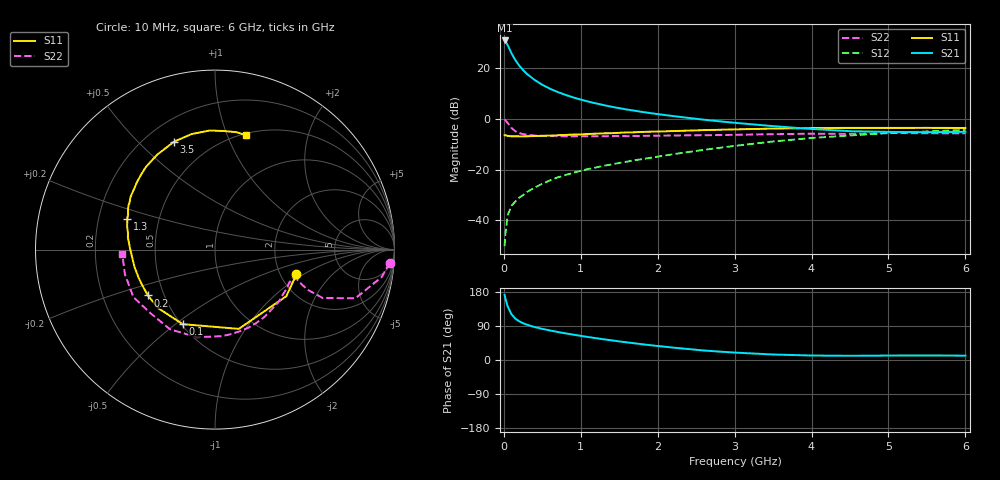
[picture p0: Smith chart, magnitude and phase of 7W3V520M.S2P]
! Infineon Technologies  Discrete & RF Semiconductors
! BFS17W
! Si NPN RF Bipolar Junction Transistor in SOT323
! VCE = 3.5 V  IC = 20 mA
! Common Emitter S-Parameters:  August  1999
# GHz  S  MA  R  50
!  f  S11  S21  S12  S22
! GHz  MAG  ANG  MAG  ANG  MAG  ANG  MAG  ANG
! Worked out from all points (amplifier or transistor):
!   36 points, 10 MHz to 6 GHz, reference 50 ohm
!   highest |S21| = 30.9 dB at 10 MHz (marker M1)
!   |S21| within 3 dB of that: start of sweep to 67.79 MHz
!   unconditionally stable (mu >= 1): 266.7 MHz to 2.291 GHz; 4.78 GHz to end of sweep
!   at 250 MHz: K = 0.98, MSG = 24.6 dB, |S12| = -30.0 dB
!   at 1.4 GHz: K = 1.19, MAG = 8.8 dB, |S12| = -18.0 dB
!   at 6 GHz: K = 1.06, MAG = -1.9 dB, |S12| = -4.4 dB
!   S11 on the Smith chart (normalised r, x): 10 MHz: 2.44, -0.86; 100 MHz: 0.51, -0.53; 200 MHz: 0.41, -0.26; 1.3 GHz: 0.33, +0.15; 3.5 GHz: 0.31, +0.64; 6 GHz: 0.52, +1.17
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0.01  0.4739 -16.8  35.02 171.4  0.0031 83.5  0.9766 -4.3
0.02  0.4749 -33.1  34.06 162.5  0.0054 81.4  0.9419 -9.3
0.05  0.4611 -73.3  28.28 141.2  0.0127 67.4  0.8281 -19.1
0.1  0.4527 -113.4  19.53 120.5  0.0194 59.1  0.6579 -24.2
0.15  0.4542 -133.9  14.31 109.1  0.0235 58.2  0.5692 -23.5
0.2  0.453 -145.7  11.19 102.1  0.0281 60.9  0.5255 -22.1
0.25  0.4514 -153.8  9.11 97.1  0.0315 61.3  0.4995 -20.7
0.3  0.4535 -159.4  7.672 93.2  0.0361 63.0  0.4865 -20.0
0.4  0.4588 -167.8  5.828 86.9  0.0443 66.2  0.4682 -19.4
0.5  0.4621 -173.3  4.692 82.1  0.0526 67.8  0.4621 -19.7
0.6  0.4675 -177.6  3.914 77.9  0.0614 68.7  0.4579 -20.6
0.7  0.4745 178.7  3.377 74.0  0.0702 69.5  0.4554 -22.1
0.9  0.4901 172.2  2.645 67.0  0.0862 70.2  0.4526 -25.7
1.1  0.5037 166.1  2.183 60.5  0.1029 70.7  0.4539 -30.2
1.3  0.5189 160.6  1.861 54.6  0.1189 70.9  0.4539 -35.3
1.6  0.5408 153.2  1.526 46.5  0.1433 71.2  0.4569 -43.2
2.2  0.5744 139.3  1.134 32.7  0.2007 71.2  0.4695 -60.8
2.8  0.6084 125.6  0.895 22.2  0.2682 68.2  0.4792 -79.5
3.5  0.643 110.8  0.718 14.5  0.3581 62.1  0.4987 -101.8
4.5  0.664 92.7  0.571 11.1  0.4701 49.0  0.5048 -135.4
5.5  0.6651 79.6  0.546 11.9  0.5649 36.2  0.5205 -164.7
6  0.6597 74.6  0.555 11.5  0.6025 30.0  0.5172 -177.5
